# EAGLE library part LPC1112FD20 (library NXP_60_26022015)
32-bit ARM Cortex-M0 microcontroller; up to 64 kB flash and 8 kB SRAM The LPC1110/11/12/13/14/15 are a ARM Cortex-M0 based, low-cost 32-bit MCU family, designed for 8/16-bit microcontroller applications, offering performance, low power, simple instruction set and memory addressing together with reduced code size compared to existing 8/16-bit architectures. The LPC1110/11/12/13/14/15 operate at CPU frequencies of up to 50 MHz. The peripheral complement of the LPC1110/11/12/13/14/15 includes up to 64 kB of flash memory, up to 8 kB of data memory, one Fast-mode Plus I 2 C-bus interface, one RS-485/EIA-485 UART, up to two SPI interfaces with SSP features, four general purpose counter/timers, a 10-bit ADC, and up to 42 general purpose I/O pins. Remark: The LPC111x series consists of the LPC1100 series (parts LPC111x/101/201/301), LPC1100L series (parts LPC111x/002/102/202/302), and the LPC1100XL series (parts LPC111x/103/203/303/323/333). The LPC1100L and LPC1100XL series include the power profiles, a windowed watchdog timer, and a configurable open-drain mode. AAL Eindhoven MK
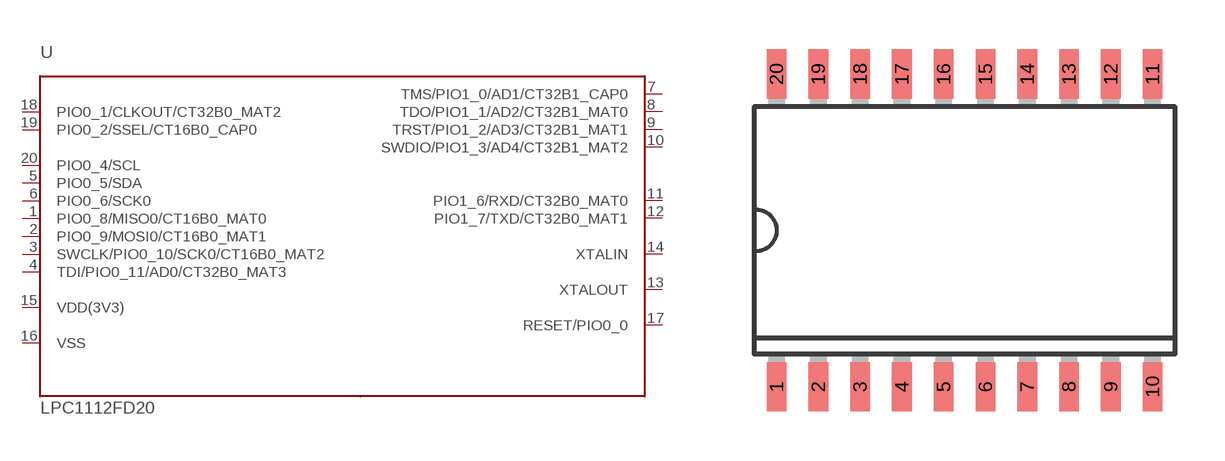
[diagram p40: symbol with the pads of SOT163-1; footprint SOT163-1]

Designator prefix U

## LPC1112FD20/102 (ADC: 5; FLASH: 16kB; GPIO: 16; PWR_PROFILES: yes; SERIES: LPC1100L; SPI: 1; SRAM: 4kB)  [SOT163-1]
1  PIO0_8/MISO0/CT16B0_MAT0
2  PIO0_9/MOSI0/CT16B0_MAT1
3  SWCLK/PIO0_10/SCK0/CT16B0_MAT2
4  TDI/PIO0_11/AD0/CT32B0_MAT3
5  PIO0_5/SDA
6  PIO0_6/SCK0
7  TMS/PIO1_0/AD1/CT32B1_CAP0
8  TDO/PIO1_1/AD2/CT32B1_MAT0
9  TRST/PIO1_2/AD3/CT32B1_MAT1
10  SWDIO/PIO1_3/AD4/CT32B1_MAT2
11  PIO1_6/RXD/CT32B0_MAT0
12  PIO1_7/TXD/CT32B0_MAT1
13  XTALOUT  out
14  XTALIN  in
15  VDD(3V3)  pwr
16  VSS  pwr
17  RESET/PIO0_0
18  PIO0_1/CLKOUT/CT32B0_MAT2
19  PIO0_2/SSEL/CT16B0_CAP0
20  PIO0_4/SCL

## Footprint SOT163-1 (pad centres in mm)
SOT163-1 SO20: plastic small outline package; 20 leads; body width 7.5 mm JEDEC: MS-013 IEC: 075E04
smd 0.6 x 1.5: 1 -5.715,-4.75; 2 -4.445,-4.75; 3 -3.175,-4.75; 4 -1.905,-4.75; 5 -0.635,-4.75; 6 0.635,-4.75; 7 1.905,-4.75; 8 3.175,-4.75; 9 4.445,-4.75; 10 5.715,-4.75; 11 5.715,4.75; 12 4.445,4.75; 13 3.175,4.75; 14 1.905,4.75; 15 0.635,4.75; 16 -0.635,4.75; 17 -1.905,4.75; 18 -3.175,4.75; 19 -4.445,4.75; 20 -5.715,4.75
